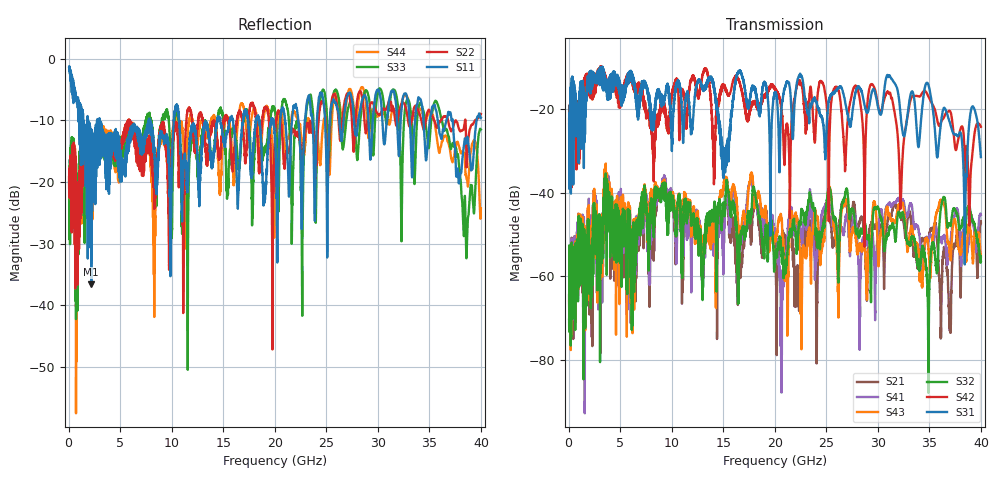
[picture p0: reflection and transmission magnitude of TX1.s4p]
!Agilent Technologies,N5245A,MY49151084,A.09.00.04
!Agilent N5245A: A.09.00.04
!Date: Thursday, January 20, 2011 08:38:49
!Correction: S11(Full 4 Port(1,2,3,4))
!S12(Full 4 Port(1,2,3,4))
!S13(Full 4 Port(1,2,3,4))
!S14(Full 4 Port(1,2,3,4))
!S21(Full 4 Port(1,2,3,4))
!S22(Full 4 Port(1,2,3,4))
!S23(Full 4 Port(1,2,3,4))
!S24(Full 4 Port(1,2,3,4))
!S31(Full 4 Port(1,2,3,4))
!S32(Full 4 Port(1,2,3,4))
!S33(Full 4 Port(1,2,3,4))
!S34(Full 4 Port(1,2,3,4))
!S41(Full 4 Port(1,2,3,4))
!S42(Full 4 Port(1,2,3,4))
!S43(Full 4 Port(1,2,3,4))
!S44(Full 4 Port(1,2,3,4))
!S4P File: Measurements: <S11,S12,S13,S14>,
!<S21,S22,S23,S24>,
!<S31,S32,S33,S34>,
!<S41,S42,S43,S44>:
# Hz S  dB  R 50
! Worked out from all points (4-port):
!   3996 points, 50 MHz to 40 GHz, reference 50 ohm
!   strongest paths, dB at 50 MHz, 10.04 GHz, 20.03 GHz, 30.02 GHz, 40 GHz:
!     S31: -23.5, -26.9, -16.0, -19.4, -31.4
!     S42: -22.3, -15.7, -15.2, -18.9, -24.2
!     S32: -70.4, -41.8, -56.2, -43.5, -56.3
!     S43: -65.9, -41.4, -50.4, -55.0, -55.2
!     S41: -64.5, -41.2, -48.5, -49.5, -45.3
!     S21: -64.7, -41.8, -53.5, -48.3, -47.1
!   lowest |S11| = -36.6 dB at 2.2 GHz (marker M1), VSWR 1.03, Z = 51.2 - j0.917 ohm
!   |S11| at or under -10 dB: 2.991 GHz to 7.802 GHz (4.81 GHz wide, 89.1 % of centre); 10.71 GHz to 14.43 GHz (3.712 GHz wide, 29.5 % of centre); 37.26 GHz to 39.58 GHz (2.318 GHz wide, 6.03 % of centre)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
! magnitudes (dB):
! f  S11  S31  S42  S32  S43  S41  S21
! 50 MHz  -1.5  -23.5  -22.3  -70.4  -65.9  -64.5  -64.7
! 2.2 GHz  -36.6  -11.3  -13.9  -64.0  -57.7  -53.4  -71.1
! 17.65 GHz  -17.8  -16.4  -19.8  -46.4  -36.0  -37.2  -50.6
! 20.67 GHz  -8.3  -19.3  -20.6  -54.8  -46.8  -67.8  -50.8
! 31.69 GHz  -6.5  -13.9  -21.8  -51.7  -47.2  -42.4  -43.0
! 36.97 GHz  -8.9  -23.0  -20.3  -47.6  -54.0  -53.0  -71.0
! 40 GHz  -9.6  -31.4  -24.2  -56.3  -55.2  -45.3  -47.1
